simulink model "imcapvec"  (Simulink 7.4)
settings: Solver=ode45  StartTime=0.0  StopTime=2.5  MaxStep=5e-4  RelTol=1e-4

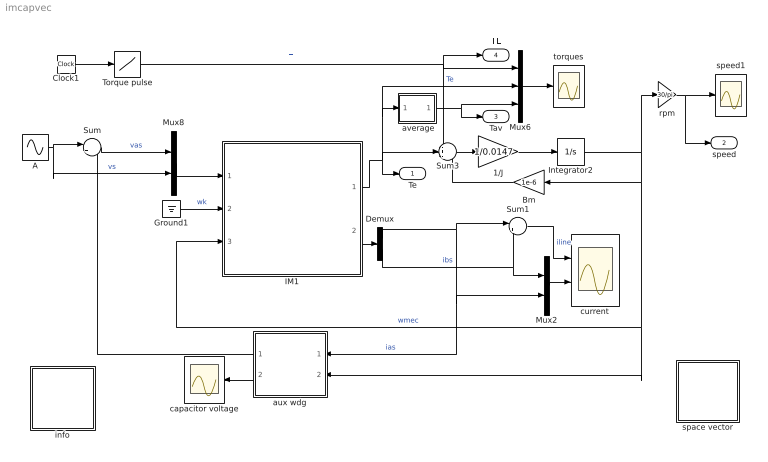
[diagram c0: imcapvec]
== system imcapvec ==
  " average" : Subsystem
  1/J : Gain  Gain=1/0.0147  ParameterDataType=sfix(16)  ParameterScaling=2^0  OutDataType=sfix(16)  OutScaling=2^0
  A : Sin  Amplitude=110*sqrt(2)  Bias=0  Frequency=2*pi*60  Phase=pi/2  Samples=10  SampleTime=0
  Bm : Gain  Gain=1e-6  ParameterDataType=sfix(16)  ParameterScaling=2^0  OutDataType=sfix(16)  OutScaling=2^0
  Clock1 : Clock
  Demux : Demux  Outputs=2
  Ground1 : Ground
  IM1 : Subsystem  mask(Inductionmachine){Rs=2.02, Rr=4.12, Lsl=8.54e-3, Lrl=3.13e-3, Lm=180e-3, wo=2*pi*60, p=4}
      mask prompts: Rs "Stator resistance [ohm]"; Rr "Rotor resistance [ohm]"; Lsl "Stator leakage inductance  [H]"; Lrl "Rotor leakage inductance [H]"; Lm "Magnetizing inductance [H]"; wo "Base frequency [rad/s]"; p "Number of poles"
      mask help: Space vector model of the induction machine in a general frame k. SI units
  Integrator2 : Integrator
  Mux2 : Mux  Inputs=2
  Mux6 : Mux  Inputs=3
  Mux8 : Mux  Inputs=2
  Sum : Sum  Inputs=|+-  OutDataType=sfix(16)  OutScaling=2^0
  Sum1 : Sum  Inputs=|++  OutDataType=sfix(16)  OutScaling=2^0
  Sum3 : Sum  Inputs=-+-  OutDataType=sfix(16)  OutScaling=2^0
  Torque pulse : Lookup  InputValues=[0 1 1 1.5 1.5 2]  Table=[0 0 2 2 3 3]  OutDataType=sfix(16)  OutScaling=2^0
  aux wdg : Subsystem  mask{Cstart=183e-6, Crun=30e-6, p=4, Nsw=3/4}
      mask prompts: Cstart "Start capacitance [F]"; Crun "Run capacitance [F}"; p "Number of poles"; Nsw "Speed when switch disconnects [pu]"
  capacitor voltage : Scope
  current : Scope  NumInputPorts=2
  info : Subsystem
  rpm : Gain  Gain=30/pi  ParameterDataType=sfix(16)  ParameterScaling=2^0  OutDataType=sfix(16)  OutScaling=2^0
  space vector : Subsystem
  speed1 : Scope
  torques : Scope
  Te : Outport
  speed : Outport  Port=2
  Tav : Outport  Port=3
  TL : Outport  Port=4
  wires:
  Sum1/1 -> current/1  "iline"
  Mux2/1 -> current/2
  Mux8/1 -> IM1/1(vs)
  Sum/1 -> Mux8/1  "vas"
  A/1 -> Sum/1, Mux8/2  "vs"
  IM1/2(is) -> Demux/1
  Demux/1 -> Sum1/1, Mux2/2, aux wdg/1(ias)  "ias"
  Demux/2 -> Sum1/2, Mux2/1  "ibs"
  1/J/1 -> Integrator2/1
  Mux6/1 -> torques/1
  Bm/1 -> Sum3/3
  Integrator2/1 -> Bm/1, aux wdg/2(wmec), IM1/3(wmec), rpm/1  "wmec"
  rpm/1 -> speed1/1, speed/1
  IM1/1(Te) -> Sum3/2, Te/1, " average"/1(sig), Mux6/2  "Te"
  Sum3/1 -> 1/J/1
  Clock1/1 -> Torque pulse/1
  Torque pulse/1 -> Mux6/1, Sum3/1, TL/1  "Tl"
  aux wdg/2(vcap) -> capacitor voltage/1
  Ground1/1 -> IM1/2(wk)  "wk"
  " average"/1(ave) -> Mux6/3, Tav/1
  aux wdg/1(vaux) -> Sum/2

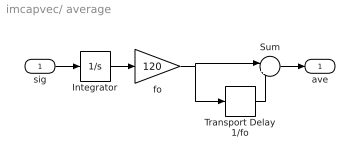
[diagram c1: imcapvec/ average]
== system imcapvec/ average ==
  sig : Inport  OutDataType=sfix(16)  OutScaling=2^0
  Integrator : Integrator
  Sum : Sum  Inputs=|+-  OutDataType=sfix(16)  OutScaling=2^0
  Transport Delay 1/fo : TransportDelay  DelayTime=1/120
  fo : Gain  Gain=120  ParameterDataType=sfix(16)  ParameterScaling=2^0  OutDataType=sfix(16)  OutScaling=2^0
  ave : Outport
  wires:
  Sum/1 -> ave/1
  Transport Delay 1/fo/1 -> Sum/2
  sig/1 -> Integrator/1
  fo/1 -> Transport Delay 1/fo/1, Sum/1
  Integrator/1 -> fo/1

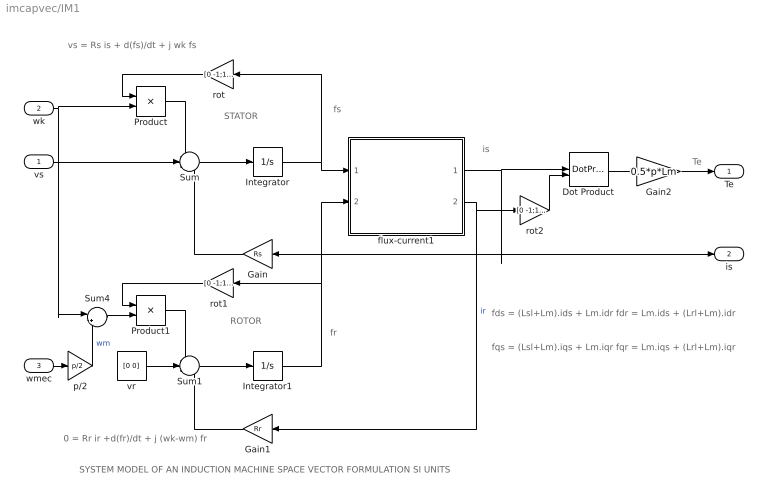
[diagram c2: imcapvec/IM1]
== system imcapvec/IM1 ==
  note: ROTOR
  note: STATOR
  note: fs
  note: is
  note: Te
  note: SYSTEM MODEL OF AN INDUCTION MACHINE SPACE VECTOR FORMULATION SI UNITS
  note: vs = Rs is + d(fs)/dt + j wk fs
  note: 0 = Rr ir +d(fr)/dt + j (wk-wm) fr
  note: fds = (Lsl+Lm).ids + Lm.idr fdr = Lm.ids + (Lrl+Lm).idr
  note: fqs = (Lsl+Lm).iqs + Lm.iqr fqr = Lm.iqs + (Lrl+Lm).iqr
  note: fr
  vs : Inport  OutDataType=sfix(16)  OutScaling=2^0
  wk : Inport  Port=2  OutDataType=sfix(16)  OutScaling=2^0
  wmec : Inport  Port=3  OutDataType=sfix(16)  OutScaling=2^0
  Dot Product : DotProduct  OutDataType=fixdt(1, 16)  OutScaling=2^-10
  Gain : Gain  Gain=Rs  ParameterDataType=sfix(16)  ParameterScaling=2^0  OutDataType=sfix(16)  OutScaling=2^0
  Gain1 : Gain  Gain=Rr  ParameterDataType=sfix(16)  ParameterScaling=2^0  OutDataType=sfix(16)  OutScaling=2^0
  Gain2 : Gain  Gain=0.5*p*Lm  ParameterDataType=sfix(16)  ParameterScaling=2^0  OutDataType=sfix(16)  OutScaling=2^0
  Integrator : Integrator  InitialCondition=[0 0]
  Integrator1 : Integrator  InitialCondition=[0 0]
  Product : Product  OutDataType=sfix(16)  OutScaling=2^0
  Product1 : Product  OutDataType=sfix(16)  OutScaling=2^0
  Sum : Sum  Inputs=-+-  OutDataType=sfix(16)  OutScaling=2^0
  Sum1 : Sum  Inputs=-+-  OutDataType=sfix(16)  OutScaling=2^0
  Sum4 : Sum  Inputs=|+-  OutDataType=sfix(16)  OutScaling=2^0
  flux-current1 : Subsystem
  p/2 : Gain  Gain=p/2  ParameterDataType=sfix(16)  ParameterScaling=2^0  OutDataType=sfix(16)  OutScaling=2^0
  rot : Gain  Gain=[0 -1;1 0]  Multiplication=Matrix(K*u)  ParameterDataType=sfix(16)  ParameterScaling=2^0  OutDataType=sfix(16)  OutScaling=2^0
  rot1 : Gain  Gain=[0 -1;1 0]  Multiplication=Matrix(K*u)  ParameterDataType=sfix(16)  ParameterScaling=2^0  OutDataType=sfix(16)  OutScaling=2^0
  rot2 : Gain  Gain=[0 -1;1 0]  Multiplication=Matrix(K*u)  ParameterDataType=sfix(16)  ParameterScaling=2^0  OutDataType=sfix(16)  OutScaling=2^0
  vr : Constant  Value=[0 0]  OutDataType=sfix(16)  OutScaling=2^0
  Te : Outport
  is : Outport  Port=2
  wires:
  Gain/1 -> Sum/3
  vr/1 -> Sum1/2
  Gain1/1 -> Sum1/3
  Integrator/1 -> flux-current1/1(fs), rot/1
  Integrator1/1 -> rot1/1, flux-current1/2(fr)
  Product1/1 -> Sum1/1
  rot1/1 -> Product1/1
  Product/1 -> Sum/1
  rot/1 -> Product/1
  Sum4/1 -> Product1/2
  vs/1 -> Sum/2
  wk/1 -> Product/2, Sum4/1
  Sum1/1 -> Integrator1/1
  Sum/1 -> Integrator/1
  flux-current1/1(is) -> Gain/1, is/1, Dot Product/1
  Dot Product/1 -> Gain2/1
  Gain2/1 -> Te/1
  wmec/1 -> p/2/1
  p/2/1 -> Sum4/2  "wm"
  rot2/1 -> Dot Product/2
  flux-current1/2(ir) -> Gain1/1, rot2/1  "ir"

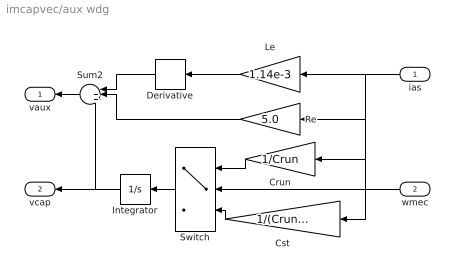
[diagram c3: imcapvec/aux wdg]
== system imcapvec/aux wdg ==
  ias : Inport  OutDataType=sfix(16)  OutScaling=2^0
  wmec : Inport  Port=2  OutDataType=sfix(16)  OutScaling=2^0
  Crun : Gain  Gain=1/Crun  ParameterDataType=sfix(16)  ParameterScaling=2^0  OutDataType=sfix(16)  OutScaling=2^0
  Cst : Gain  Gain=1/(Crun+Cstart)  ParameterDataType=sfix(16)  ParameterScaling=2^0  OutDataType=sfix(16)  OutScaling=2^0
  Derivative : Derivative
  Integrator : Integrator
  Le : Gain  Gain=1.14e-3  ParameterDataType=sfix(16)  ParameterScaling=2^0  OutDataType=sfix(16)  OutScaling=2^0
  Re : Gain  Gain=5.0  ParameterDataType=sfix(16)  ParameterScaling=2^0  OutDataType=sfix(16)  OutScaling=2^0
  Sum2 : Sum  Inputs=|+++  OutDataType=sfix(16)  OutScaling=2^0
  Switch : Switch  Threshold=Nsw*377*2/p
  vaux : Outport
  vcap : Outport  Port=2
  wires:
  Le/1 -> Derivative/1
  Derivative/1 -> Sum2/1
  Re/1 -> Sum2/2
  Cst/1 -> Switch/3
  Crun/1 -> Switch/1
  Switch/1 -> Integrator/1
  Sum2/1 -> vaux/1
  Integrator/1 -> Sum2/3, vcap/1
  wmec/1 -> Switch/2
  ias/1 -> Cst/1, Crun/1, Re/1, Le/1

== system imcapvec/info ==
  note: This demo simulates the starting characteristics of a capacitor- start capacitor-run single-phase induction motor. An abc phase variable version of this case is given in file

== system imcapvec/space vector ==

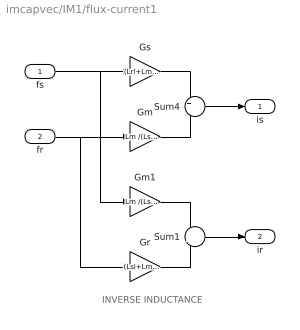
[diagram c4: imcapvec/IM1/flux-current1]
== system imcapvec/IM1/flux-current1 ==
  note: INVERSE INDUCTANCE
  fs : Inport  OutDataType=sfix(16)  OutScaling=2^0
  fr : Inport  Port=2  OutDataType=sfix(16)  OutScaling=2^0
  Gm : Gain  Gain=Lm /(Lsl*Lrl+Lsl*Lm+Lrl*Lm)  ParameterDataType=sfix(16)  ParameterScaling=2^0  OutDataType=sfix(16)  OutScaling=2^0
  Gm1 : Gain  Gain=Lm /(Lsl*Lrl+Lsl*Lm+Lrl*Lm)  ParameterDataType=sfix(16)  ParameterScaling=2^0  OutDataType=sfix(16)  OutScaling=2^0
  Gr : Gain  Gain=(Lsl+Lm )/(Lsl*Lrl+Lsl*Lm+Lrl*Lm)  ParameterDataType=sfix(16)  ParameterScaling=2^0  OutDataType=sfix(16)  OutScaling=2^0
  Gs : Gain  Gain=(Lrl+Lm) /(Lsl*Lrl+Lsl*Lm+Lrl*Lm)  ParameterDataType=sfix(16)  ParameterScaling=2^0  OutDataType=sfix(16)  OutScaling=2^0
  Sum1 : Sum  Inputs=-+  OutDataType=sfix(16)  OutScaling=2^0
  Sum4 : Sum  Inputs=+-  OutDataType=sfix(16)  OutScaling=2^0
  is : Outport
  ir : Outport  Port=2
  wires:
  fs/1 -> Gs/1, Gm1/1
  Gs/1 -> Sum4/1
  fr/1 -> Gm/1, Gr/1
  Gm/1 -> Sum4/2
  Sum4/1 -> is/1
  Gm1/1 -> Sum1/1
  Gr/1 -> Sum1/2
  Sum1/1 -> ir/1
